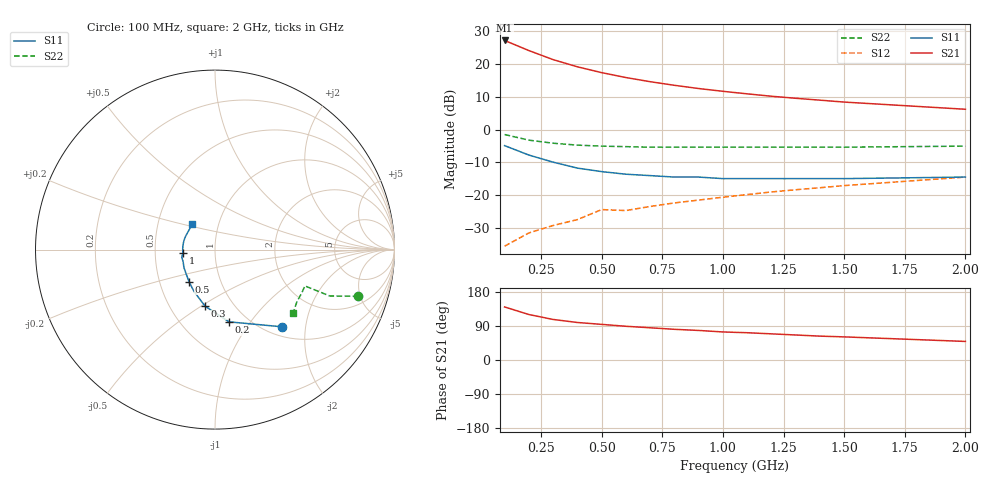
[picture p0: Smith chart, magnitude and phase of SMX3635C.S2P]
! HSMX-3635 Common Emitter
! Vce=10V Ic=15 ma
# ghz s ma r 50
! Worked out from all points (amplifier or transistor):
!   16 points, 100 MHz to 2 GHz, reference 50 ohm
!   highest |S21| = 27.0 dB at 100 MHz (marker M1)
!   |S21| within 3 dB of that: start of sweep to 197.8 MHz
!   unconditionally stable (mu >= 1): 595.3 MHz to 1.652 GHz
!   at 300 MHz: K = 0.80, MSG = 25.2 dB, |S12| = -29.1 dB
!   at 900 MHz: K = 1.04, MAG = 15.7 dB, |S12| = -21.4 dB
!   at 2 GHz: K = 0.96, MSG = 10.3 dB, |S12| = -14.4 dB
!   S11 on the Smith chart (normalised r, x): 100 MHz: 1.17, -1.49; 200 MHz: 0.82, -0.80; 300 MHz: 0.74, -0.52; 500 MHz: 0.71, -0.27; 1 GHz: 0.70, -0.03; 2 GHz: 0.75, +0.22
0.1  0.57 -49.0  22.46 140.0  0.017 70.0  0.84 -18.0
0.2  0.41 -79.0  15.78 120.0  0.027 66.0  0.69 -22.0
0.3  0.32 -100.0  11.5 107.0  0.035 67.0  0.62 -22.0
0.4  0.26 -117.0  8.95 99.0  0.043 69.0  0.58 -22.0
0.5  0.23 -129.0  7.3 94.0  0.061 70.0  0.56 -22.0
0.6  0.21 -140.0  6.15 89.0  0.059 72.0  0.55 -22.0
0.7  0.2 -150.0  5.32 85.0  0.068 73.0  0.54 -22.0
0.8  0.19 -159.0  4.69 81.0  0.077 74.0  0.54 -23.0
0.9  0.19 -167.0  4.19 78.0  0.085 74.0  0.54 -25.0
1  0.18 -174.0  3.8 74.0  0.094 74.0  0.54 -26.0
1.1  0.18 179.0  3.48 72.0  0.103 74.0  0.54 -27.0
1.2  0.18 173.0  3.2 69.0  0.113 74.0  0.54 -28.0
1.3  0.18 167.0  2.98 66.0  0.122 74.0  0.54 -30.0
1.4  0.18 162.0  2.79 63.0  0.131 74.0  0.54 -31.0
1.5  0.18 156.0  2.61 61.0  0.141 73.0  0.54 -32.0
2  0.19 132.0  2.03 49.0  0.19 71.0  0.56 -39.0
